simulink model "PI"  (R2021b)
settings: Solver=VariableStepAuto  StartTime=0.0  StopTime=5  RelTol=1e-3
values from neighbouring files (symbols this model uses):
  a = 0.27    [CompareGazeboSimulink.m]    (also in RobotModel.m)
  b = 0.31    [CompareGazeboSimulink.m]    (also in RobotModel.m)
  desired_ang = 1    [RobotModel.m]
  desired_vel = 2    [RobotModel.m]
  Dflag = 1    [RobotModel.m]
  distAng = 0    [RobotModel.m]
  distVel = 0    [RobotModel.m]
  fro = 0.02    [CompareGazeboSimulink.m]    (also in RobotModel.m)
  fsl = 0.8    [CompareGazeboSimulink.m]    (also in RobotModel.m)
  fsly = 0.8    [CompareGazeboSimulink.m]    (also in RobotModel.m)
  I = (1/12)*m*((2*t)^2 + 0.12^2) + 1.5    (= 2.384)    [CompareGazeboSimulink.m]    (also in RobotModel.m = 0.866666666667)
  Iflag = 1    [RobotModel.m]
  K = 22    [RobotModel.m]
  ko = 0    [CompareGazeboSimulink.m]    (also in RobotModel.m = 0.25)
  kt = 0.58    [CompareGazeboSimulink.m]    (also in RobotModel.m)
  m = 51    [CompareGazeboSimulink.m]    (also in RobotModel.m = 50)
  mdy = 10    [CompareGazeboSimulink.m]    (also in RobotModel.m)
  mst = 10    [CompareGazeboSimulink.m]    (also in RobotModel.m)
  N = 0    [RobotModel.m]
  r = 0.19    [CompareGazeboSimulink.m]    (also in RobotModel.m)
  T_vel_variance = 0.0005    [RobotModel.m]
  Td = 0.0125    [RobotModel.m]
  Th0 = 0    [CompareGazeboSimulink.m]    (also in RobotModel.m = 0.9714)
  Th_vel0 = 0    [CompareGazeboSimulink.m]    (also in RobotModel.m)
  Ti = 0.1    [RobotModel.m]
  Ts = 0.01    [CompareGazeboSimulink.m]    (also in RobotModel.m = 0.05)
  X0 = 0    [CompareGazeboSimulink.m]    (also in RobotModel.m)
  x_vel0 = 0    [CompareGazeboSimulink.m]    (also in RobotModel.m)
  x_vel_variance = 0.0005    [RobotModel.m]
  Y0 = 0    [CompareGazeboSimulink.m]    (also in RobotModel.m = 2.5)

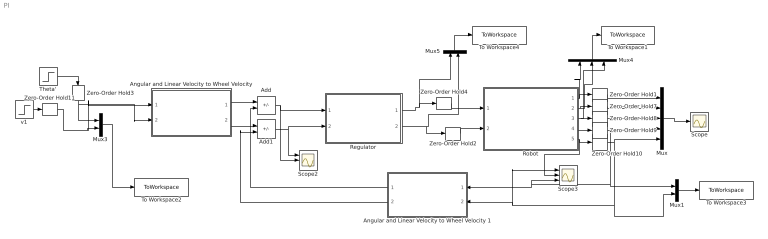
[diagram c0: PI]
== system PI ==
  Add : Sum  Inputs=+-
  Add1 : Sum  Inputs=+-
  Angular and Linear Velocity to Wheel Velocity : Subsystem
  Angular and Linear Velocity to Wheel Velocity 1 : Subsystem
  Mux : Mux  Inputs=5
  Mux1 : Mux  Inputs=2
  Mux3 : Mux  Inputs=2
  Mux4 : Mux  Inputs=3
  Mux5 : Mux  Inputs=2
  Regulator : Subsystem
  Robot : Subsystem
  Scope : Scope
  Scope2 : Scope  NumInputPorts=3
  Scope3 : Scope  NumInputPorts=3
  Theta' : Step  After=desired_ang  SampleTime=0
  To Workspace1 : ToWorkspace  VariableName=ActualPos  SaveFormat=Timeseries  SampleTime=-1
  To Workspace2 : ToWorkspace  VariableName=DesiredVel  SaveFormat=Timeseries  SampleTime=-1
  To Workspace3 : ToWorkspace  VariableName=ActualVel  SaveFormat=Timeseries  SampleTime=-1
  To Workspace4 : ToWorkspace  VariableName=Forces  SaveFormat=Timeseries  SampleTime=-1
  Zero-Order Hold{1..4,7..11} (9 alike) : ZeroOrderHold  SampleTime=Ts
  v1 : Step  After=desired_vel  SampleTime=0
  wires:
  Zero-Order Hold3/1 -> Mux3/1, Angular and Linear Velocity to Wheel Velocity/2(Angular Velocity)
  Zero-Order Hold11/1 -> Angular and Linear Velocity to Wheel Velocity/1(Linear Velocity), Mux3/2
  Zero-Order Hold2/1 -> Robot/2(Right Force)
  Zero-Order Hold4/1 -> Robot/1(Left Force)
  Robot/5(v) -> Scope3/2, Zero-Order Hold10/1
  Robot/3(Theta) -> Mux4/3, Zero-Order Hold8/1
  Robot/2(Y) -> Mux4/2, Zero-Order Hold7/1
  v1/1 -> Zero-Order Hold11/1
  Mux5/1 -> To Workspace4/1
  Mux1/1 -> To Workspace3/1
  Regulator/2(Right force action) -> Mux5/2, Zero-Order Hold2/1
  Add/1 -> Scope2/2, Regulator/1(wl)
  Angular and Linear Velocity to Wheel Velocity/2("wr ") -> Add1/1
  Robot/1(X) -> Mux4/1, Zero-Order Hold1/1
  Angular and Linear Velocity to Wheel Velocity/1(wl) -> Add/1
  Zero-Order Hold8/1 -> Mux/3
  Robot/4(Theta') -> Zero-Order Hold9/1
  Mux3/1 -> To Workspace2/1
  Add1/1 -> Scope2/1, Regulator/2(wr)
  Mux4/1 -> To Workspace1/1
  Angular and Linear Velocity to Wheel Velocity 1/2("wr ") -> Add1/2
  Zero-Order Hold1/1 -> Mux/1
  Zero-Order Hold7/1 -> Mux/2
  Zero-Order Hold10/1 -> Mux1/2, Scope3/1, Angular and Linear Velocity to Wheel Velocity 1/2(Linear Velocity), Mux/5
  Angular and Linear Velocity to Wheel Velocity 1/1(wl) -> Add/2
  Zero-Order Hold9/1 -> Mux1/1, Scope3/3, Angular and Linear Velocity to Wheel Velocity 1/1(Angular Velocity), Mux/4
  Regulator/1(Left Force action) -> Mux5/1, Zero-Order Hold4/1
  Theta'/1 -> Zero-Order Hold3/1
  Mux/1 -> Scope/1

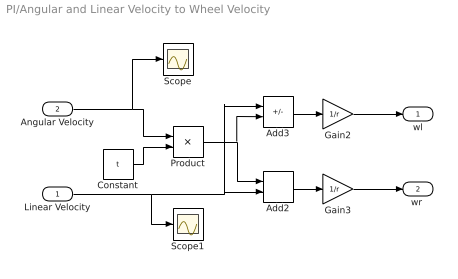
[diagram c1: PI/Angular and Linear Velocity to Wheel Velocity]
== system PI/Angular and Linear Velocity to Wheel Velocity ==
  Linear Velocity : Inport
  Angular Velocity : Inport  Port=2
  Add2 : Sum
  Add3 : Sum  Inputs=+-
  Constant : Constant  Value=t
  Gain2 : Gain  Gain=1/r
  Gain3 : Gain  Gain=1/r
  Product : Product
  Scope : Scope
  Scope1 : Scope
  wl : Outport
  "wr " : Outport  Port=2
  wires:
  Gain2/1 -> wl/1
  Linear Velocity/1 -> Scope1/1, Add2/2, Add3/1
  Gain3/1 -> "wr "/1
  Product/1 -> Add3/2, Add2/1
  Constant/1 -> Product/2
  Add3/1 -> Gain2/1
  Add2/1 -> Gain3/1
  Angular Velocity/1 -> Scope/1, Product/1

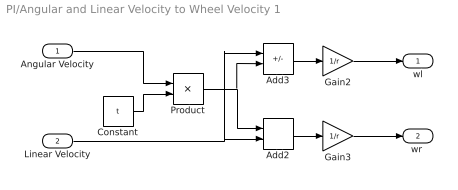
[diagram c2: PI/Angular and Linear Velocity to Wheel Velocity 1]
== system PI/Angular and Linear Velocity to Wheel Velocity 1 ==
  Angular Velocity : Inport
  Linear Velocity : Inport  Port=2
  Add2 : Sum
  Add3 : Sum  Inputs=+-
  Constant : Constant  Value=t
  Gain2 : Gain  Gain=1/r
  Gain3 : Gain  Gain=1/r
  Product : Product
  wl : Outport
  "wr " : Outport  Port=2
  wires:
  Angular Velocity/1 -> Product/1
  Add2/1 -> Gain3/1
  Add3/1 -> Gain2/1
  Constant/1 -> Product/2
  Product/1 -> Add2/1, Add3/2
  Gain3/1 -> "wr "/1
  Linear Velocity/1 -> Add3/1, Add2/2
  Gain2/1 -> wl/1

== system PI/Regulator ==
  wl : Inport
  wr : Inport  Port=2
  PSDN : Subsystem
  PSDN1 : Subsystem
  Left Force action : Outport
  Right force action : Outport  Port=2
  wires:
  wl/1 -> PSDN/1(wl)
  PSDN/1(Left Force action) -> Left Force action/1
  wr/1 -> PSDN1/1(wr)
  PSDN1/1(Right force action) -> Right force action/1

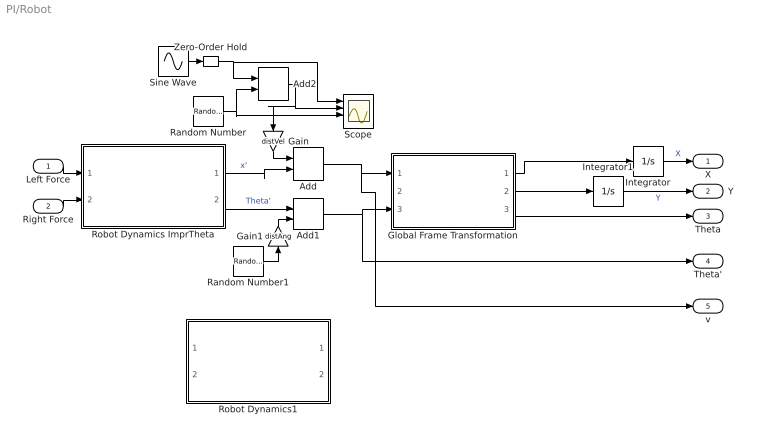
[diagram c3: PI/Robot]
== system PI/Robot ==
  Left Force : Inport
  Right Force : Inport  Port=2
  Add : Sum
  Add1 : Sum
  Add2 : Sum
  Gain : Gain  Gain=distVel
  Gain1 : Gain  Gain=distAng
  Global Frame Transformation : Subsystem
  Integrator : Integrator  InitialCondition=X0
  Integrator1 : Integrator  InitialCondition=Y0
  Random Number : RandomNumber  Variance=x_vel_variance  SampleTime=0.2
  Random Number1 : RandomNumber  Variance=T_vel_variance  SampleTime=0.2
  Robot Dynamics ImprTheta : Subsystem
  Robot Dynamics1 : Subsystem  Commented=on
  Scope : Scope  NumInputPorts=4
  Sine Wave : Sin  Amplitude=0.1*desired_vel  Frequency=0.5  SampleTime=0
  Zero-Order Hold : ZeroOrderHold  SampleTime=0.25
  X : Outport
  Y : Outport  Port=2
  Theta : Outport  Port=3
  Theta' : Outport  Port=4
  v : Outport  Port=5
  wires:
  Random Number/1 -> Add2/2, Scope/3
  Add2/1 -> Gain/1, Scope/2
  Gain/1 -> Add/1
  Sine Wave/1 -> Zero-Order Hold/1
  Add/1 -> v/1, Global Frame Transformation/1(x')
  Add1/1 -> Theta'/1, Global Frame Transformation/3(Theta')
  Random Number1/1 -> Gain1/1
  Left Force/1 -> Robot Dynamics ImprTheta/1(Left Force)
  Gain1/1 -> Add1/2
  Integrator1/1 -> Y/1  "Y"
  Zero-Order Hold/1 -> Scope/1, Add2/1
  Robot Dynamics ImprTheta/1(x') -> Add/2  "x'"
  Global Frame Transformation/2(Y') -> Integrator1/1
  Integrator/1 -> X/1  "X"
  Right Force/1 -> Robot Dynamics ImprTheta/2(Right Force)
  Global Frame Transformation/1(X') -> Integrator/1
  Global Frame Transformation/3(Theta) -> Theta/1
  Robot Dynamics ImprTheta/2(Theta') -> Add1/1  "Theta'"

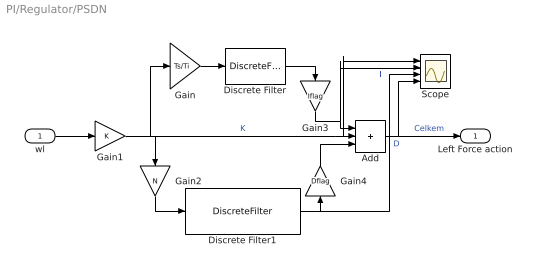
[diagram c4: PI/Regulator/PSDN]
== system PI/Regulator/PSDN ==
  wl : Inport
  Add : Sum  Inputs=3
  Discrete Filter : DiscreteFilter  Numerator=[0 1]  Denominator=[1 -1]
  Discrete Filter1 : DiscreteFilter  Numerator=[1 -1]  Denominator=[1 -exp(-Ts*N/Td)]
  Gain : Gain  Gain=Ts/Ti
  Gain1 : Gain  Gain=K
  Gain2 : Gain  Gain=N
  Gain3 : Gain  Gain=Iflag
  Gain4 : Gain  Gain=Dflag
  Scope : Scope  NumInputPorts=4
  Left Force action : Outport
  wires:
  Discrete Filter/1 -> Gain3/1
  Discrete Filter1/1 -> Scope/3, Gain4/1  "D"
  wl/1 -> Gain1/1
  Add/1 -> Left Force action/1, Scope/4  "Celkem"
  Gain/1 -> Discrete Filter/1
  Gain1/1 -> Gain2/1, Gain/1, Scope/1, Add/2  "K"
  Gain2/1 -> Discrete Filter1/1
  Gain3/1 -> Scope/2, Add/1  "I"
  Gain4/1 -> Add/3

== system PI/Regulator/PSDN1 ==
  wr : Inport
  Add : Sum  Inputs=3
  Discrete Filter : DiscreteFilter  Numerator=[0 1]  Denominator=[1 -1]
  Discrete Filter1 : DiscreteFilter  Numerator=[1 -1]  Denominator=[1 -exp(-Ts*N/Td)]
  Gain : Gain  Gain=Ts/Ti
  Gain1 : Gain  Gain=K
  Gain2 : Gain  Gain=N
  Gain3 : Gain  Gain=Iflag
  Gain4 : Gain  Gain=Dflag
  Right force action : Outport
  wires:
  Gain2/1 -> Discrete Filter1/1
  Gain1/1 -> Add/2, Gain/1, Gain2/1
  Gain/1 -> Discrete Filter/1
  Add/1 -> Right force action/1
  wr/1 -> Gain1/1
  Discrete Filter1/1 -> Gain4/1
  Discrete Filter/1 -> Gain3/1
  Gain3/1 -> Add/1
  Gain4/1 -> Add/3

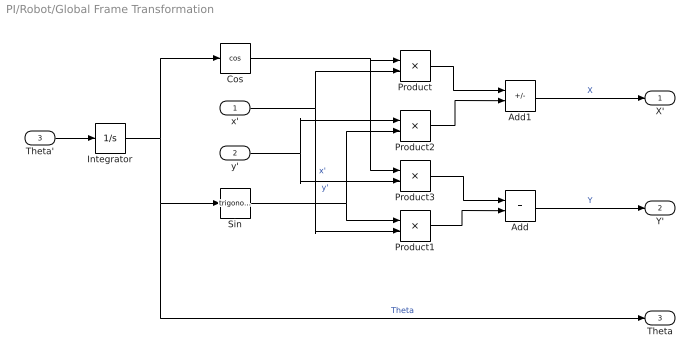
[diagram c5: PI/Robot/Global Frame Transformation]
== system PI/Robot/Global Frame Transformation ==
  x' : Inport
  y' : Inport  Port=2
  Theta' : Inport  Port=3
  Add : Sum
  Add1 : Sum  Inputs=+-
  Cos : Trigonometry  Operator=cos
  Integrator : Integrator  InitialCondition=Th0
  Product{,1..3} (4 alike) : Product
  Sin : Trigonometry
  X' : Outport
  Y' : Outport  Port=2
  Theta : Outport  Port=3
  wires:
  Add/1 -> Y'/1  "Y"
  Integrator/1 -> Theta/1, Sin/1, Cos/1  "Theta"
  Product1/1 -> Add/2
  x'/1 -> Product/2, Product1/2  "x'"
  Sin/1 -> Product1/1, Product2/2
  Product2/1 -> Add1/2
  Product3/1 -> Add/1
  Product/1 -> Add1/1
  Cos/1 -> Product/1, Product3/1
  y'/1 -> Product3/2, Product2/1  "y'"
  Add1/1 -> X'/1  "X"
  Theta'/1 -> Integrator/1

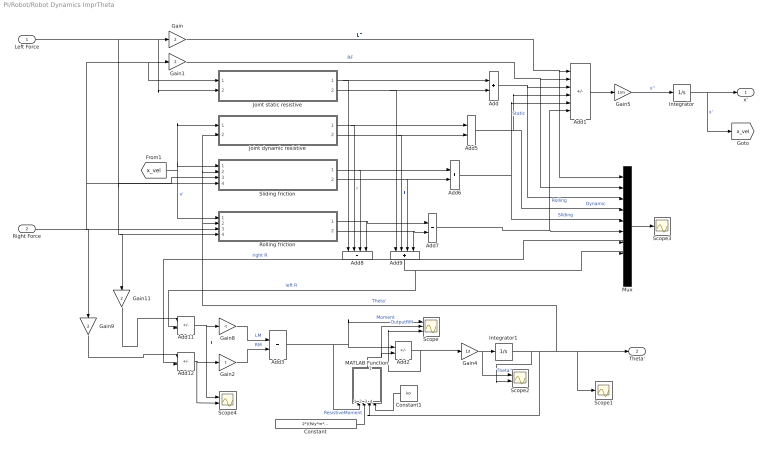
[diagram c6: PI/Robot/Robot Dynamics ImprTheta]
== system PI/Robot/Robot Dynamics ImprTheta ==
  Left Force : Inport
  Right Force : Inport  Port=2
  Add{,3,5..7} (5 alike) : Sum
  Add1 : Sum  Inputs=++----
  Add11 : Sum  Inputs=+-
  Add12 : Sum  Inputs=+-
  Add2 : Sum  Inputs=+-
  Add8 : Sum  Inputs=++++
  Add9 : Sum  Inputs=++++
  Constant : Constant  Value=2*((fsly*m*9.81)/(a+b))*a*b*kt
  Constant1 : Constant  Value=ko
  Gain{,1,9,11} (4 alike) : Gain  Gain=2
  Gain2 : Gain  Gain=t
  Gain4 : Gain  Gain=1/I
  Gain5 : Gain  Gain=1/m
  Gain8 : Gain  Gain=-t
  Integrator : Integrator  InitialCondition=x_vel0
  Integrator1 : Integrator  InitialCondition=Th_vel0
  Joint dynamic resistive : Subsystem
  Joint static resistive : Subsystem
  MATLAB Function : MATLAB Function  TreatAsAtomicUnit=on
  Mux : Mux  Inputs=10
  Rolling friction : Subsystem
  Scope : Scope  NumInputPorts=3
  Scope1 : Scope
  Scope2 : Scope  NumInputPorts=2
  Scope3 : Scope
  Scope4 : Scope  NumInputPorts=2
  Sliding friction : Subsystem
  x' : Outport
  Theta' : Outport  Port=2
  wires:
  Gain4/1 -> Scope2/1, Integrator1/1  "Theta''"
  Integrator1/1 -> Scope2/2, Sliding friction/2(Theta'), Joint dynamic resistive/2(Theta'), Rolling friction/2(Theta'), Scope1/1, Theta'/1, MATLAB Function/3(Omega)  "Theta'"
  Gain1/1 -> Mux/2, Add1/2  "RF"
  Add1/1 -> Gain5/1
  Gain5/1 -> Integrator/1  "x''"
  Integrator/1 -> x'/1, [x_vel]  "x'"
  [x_vel] -> Joint dynamic resistive/1("Local Long Velocity "), Sliding friction/1(Local longitudal velocity), Rolling friction/1(Local longitudal velocity)  "x'"
  Joint static resistive/2(Static Resistive Force Left) -> Add9/1, Add/2
  Joint dynamic resistive/1(Dynamic Resistive Force Right) -> Add8/2, Add5/1  "r"
  Joint dynamic resistive/2(Dynamic Resistive Force Left) -> Add9/2, Add5/2  "l"
  Sliding friction/1(Friction Right Force) -> Add8/3, Add6/1
  Sliding friction/2(Friction Left Force) -> Add9/3, Add6/2
  Rolling friction/1(Friction Right Force) -> Add8/4, Add7/1
  Rolling friction/2(Friction Left Force) -> Add9/4, Add7/2
  Add/1 -> Add1/3, Mux/3  "Static"
  Add6/1 -> Add1/5, Mux/5  "Sliding"
  Add7/1 -> Mux/6, Add1/6  "Rolling"
  Add5/1 -> Mux/4, Add1/4  "Dynamic"
  Add9/1 -> Add11/2, Mux/8  "left R"
  Add8/1 -> Add12/2, Mux/7  "right R"
  Mux/1 -> Scope3/1
  Add11/1 -> Scope4/1, Gain8/1  "LL"
  Add12/1 -> Scope4/2, Gain2/1
  Gain9/1 -> Add12/1
  Gain11/1 -> Add11/1
  Gain8/1 -> Add3/1  "LM"
  Gain2/1 -> Add3/2  "RM"
  Gain/1 -> Mux/1, Add1/1  "LF"
  Joint static resistive/1(Static Resistive Force Right) -> Add8/1, Add/1
  Add2/1 -> Scope/3, Gain4/1
  Add3/1 -> Scope/1, Add2/1, MATLAB Function/1(Moment)  "Moment"
  MATLAB Function/1(y) -> Scope/2, Add2/2  "OutputRM"
  Constant/1 -> MATLAB Function/2(ResistiveMoment)  "ResistiveMoment"
  Left Force/1 -> Gain11/1, Rolling friction/4(Fl), Sliding friction/4(Fl), Joint static resistive/2("Fl "), Gain/1
  Right Force/1 -> Gain9/1, Rolling friction/3(Fr), Sliding friction/3(Fr), Joint static resistive/1(Fr), Gain1/1
  Constant1/1 -> MATLAB Function/4(ko)

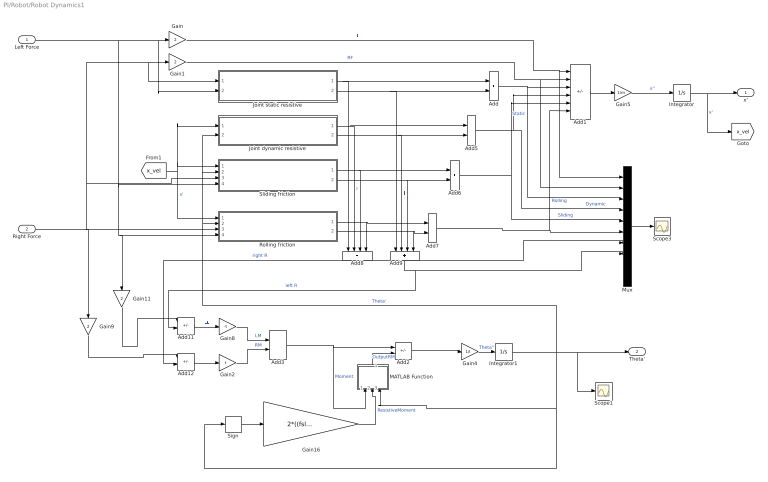
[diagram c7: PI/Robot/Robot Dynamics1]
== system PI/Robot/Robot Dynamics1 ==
  Left Force : Inport
  Right Force : Inport  Port=2
  Add{,3,5..7} (5 alike) : Sum
  Add1 : Sum  Inputs=++----
  Add11 : Sum  Inputs=+-
  Add12 : Sum  Inputs=+-
  Add2 : Sum  Inputs=+-
  Add8 : Sum  Inputs=++++
  Add9 : Sum  Inputs=++++
  Gain{,1,9,11} (4 alike) : Gain  Gain=2
  Gain16 : Gain  Gain=2*((fsly*m*9.81)/(a+b))*a*b
  Gain2 : Gain  Gain=t
  Gain4 : Gain  Gain=1/I
  Gain5 : Gain  Gain=1/m
  Gain8 : Gain  Gain=-t
  Integrator : Integrator  InitialCondition=x_vel0
  Integrator1 : Integrator  InitialCondition=Th_vel0
  Joint dynamic resistive : Subsystem
  Joint static resistive : Subsystem
  MATLAB Function : MATLAB Function  TreatAsAtomicUnit=on
  Mux : Mux  Inputs=10
  Rolling friction : Subsystem
  Scope1 : Scope
  Scope3 : Scope
  Sign : Signum
  Sliding friction : Subsystem
  x' : Outport
  Theta' : Outport  Port=2
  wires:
  Right Force/1 -> Rolling friction/3(Fr), Sliding friction/3(Fr), Joint static resistive/1(Fr), Gain1/1, Gain9/1
  Gain4/1 -> Integrator1/1  "Theta''"
  Integrator1/1 -> Sliding friction/2(Theta'), Joint dynamic resistive/2(Theta'), Rolling friction/2(Theta'), MATLAB Function/3(Omega), Sign/1, Scope1/1, Theta'/1  "Theta'"
  Left Force/1 -> Rolling friction/4(Fl), Gain11/1, Sliding friction/4(Fl), Joint static resistive/2("Fl "), Gain/1
  Gain1/1 -> Mux/2, Add1/2  "RF"
  Add1/1 -> Gain5/1
  Gain5/1 -> Integrator/1  "x''"
  Integrator/1 -> x'/1, [x_vel]  "x'"
  [x_vel] -> Joint dynamic resistive/1("Local Long Velocity "), Sliding friction/1(Local longitudal velocity), Rolling friction/1(Local longitudal velocity)  "x'"
  Joint static resistive/2(Static Resistive Force Left) -> Add9/1, Add/2
  Joint dynamic resistive/1(Dynamic Resistive Force Right) -> Add8/2, Add5/1  "r"
  Joint dynamic resistive/2(Dynamic Resistive Force Left) -> Add9/2, Add5/2  "l"
  Sliding friction/1(Friction Right Force) -> Add8/3, Add6/1
  Sliding friction/2(Friction Left Force) -> Add9/3, Add6/2
  Rolling friction/1(Friction Right Force) -> Add8/4, Add7/1
  Rolling friction/2(Friction Left Force) -> Add9/4, Add7/2
  Add/1 -> Add1/3, Mux/3  "Static"
  Add6/1 -> Add1/5, Mux/5  "Sliding"
  Add7/1 -> Mux/6, Add1/6  "Rolling"
  Add5/1 -> Mux/4, Add1/4  "Dynamic"
  Add9/1 -> Add11/2, Mux/8  "left R"
  Add8/1 -> Add12/2, Mux/7  "right R"
  Mux/1 -> Scope3/1
  Add11/1 -> Gain8/1  "LL"
  Add12/1 -> Gain2/1
  Gain9/1 -> Add12/1
  Gain11/1 -> Add11/1
  Gain8/1 -> Add3/1  "LM"
  Gain2/1 -> Add3/2  "RM"
  Gain/1 -> Mux/1, Add1/1  "LF"
  Joint static resistive/1(Static Resistive Force Right) -> Add8/1, Add/1
  Sign/1 -> Gain16/1
  Add2/1 -> Gain4/1
  Add3/1 -> Add2/1, MATLAB Function/1(Moment)  "Moment"
  MATLAB Function/1(y) -> Add2/2  "OutputRM"
  Gain16/1 -> MATLAB Function/2(ResistiveMoment)  "ResistiveMoment"

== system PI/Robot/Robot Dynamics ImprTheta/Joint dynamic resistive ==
  "Local Long Velocity " : Inport
  Theta' : Inport  Port=2
  Add2 : Sum  Inputs=+-
  Add5 : Sum
  Gain : Gain  Gain=(2*mdy)/(r*r)
  Gain1 : Gain  Gain=(2*mdy)/(r*r)
  Gain4 : Gain  Gain=t
  Scope : Scope  NumInputPorts=3
  Dynamic Resistive Force Right : Outport
  Dynamic Resistive Force Left : Outport  Port=2
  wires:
  Gain/1 -> Dynamic Resistive Force Right/1
  Gain1/1 -> Dynamic Resistive Force Left/1
  Gain4/1 -> Add5/2, Add2/2
  Theta'/1 -> Scope/3, Gain4/1
  Add5/1 -> Scope/2, Gain/1  "vr"
  Add2/1 -> Scope/1, Gain1/1  "vl"
  "Local Long Velocity "/1 -> Add2/1, Add5/1

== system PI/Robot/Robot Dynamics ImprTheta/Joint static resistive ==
  Fr : Inport
  "Fl " : Inport  Port=2
  Fsj : Gain  Gain=2*(mst/r)
  Fsj . : Gain  Gain=2*(mst/r)
  Gain1 : Gain  Gain=1/(mst/r)
  Gain2 : Gain  Gain=1/(mst/r)
  Tanh : Trigonometry  Operator=tanh
  Tanh1 : Trigonometry  Operator=tanh
  Static Resistive Force Right : Outport
  Static Resistive Force Left : Outport  Port=2
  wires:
  Fr/1 -> Gain1/1
  "Fl "/1 -> Gain2/1
  Tanh/1 -> Fsj/1
  Tanh1/1 -> Fsj ./1
  Gain1/1 -> Tanh/1
  Gain2/1 -> Tanh1/1
  Fsj/1 -> Static Resistive Force Right/1
  Fsj ./1 -> Static Resistive Force Left/1

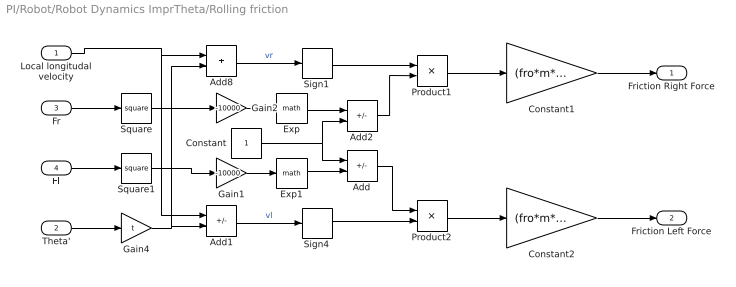
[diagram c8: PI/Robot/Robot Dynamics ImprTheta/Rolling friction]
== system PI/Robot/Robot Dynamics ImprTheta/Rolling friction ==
  Local longitudal velocity : Inport
  Theta' : Inport  Port=2
  Fr : Inport  Port=3
  Fl : Inport  Port=4
  Add : Sum  Inputs=+-
  Add1 : Sum  Inputs=+-
  Add2 : Sum  Inputs=-+
  Add8 : Sum
  Constant : Constant
  Constant1 : Gain  Gain=(fro*m*9.81)/2
  Constant2 : Gain  Gain=(fro*m*9.81)/2
  Exp : Math
  Exp1 : Math
  Gain1 : Gain  Gain=-10000
  Gain2 : Gain  Gain=-10000
  Gain4 : Gain  Gain=t
  Product1 : Product
  Product2 : Product
  Sign1 : Signum
  Sign4 : Signum
  Square : Math  Operator=square
  Square1 : Math  Operator=square
  Friction Right Force : Outport
  Friction Left Force : Outport  Port=2
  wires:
  Sign1/1 -> Product1/1
  Sign4/1 -> Product2/2
  Add8/1 -> Sign1/1  "vr"
  Fl/1 -> Square1/1
  Fr/1 -> Square/1
  Square1/1 -> Gain1/1
  Gain4/1 -> Add1/2, Add8/2
  Theta'/1 -> Gain4/1
  Add1/1 -> Sign4/1  "vl"
  Square/1 -> Gain2/1
  Gain2/1 -> Exp/1
  Gain1/1 -> Exp1/1
  Add2/1 -> Product1/2
  Add/1 -> Product2/1
  Exp1/1 -> Add/2
  Exp/1 -> Add2/1
  Constant/1 -> Add2/2, Add/1
  Local longitudal velocity/1 -> Add1/1, Add8/1
  Product1/1 -> Constant1/1
  Product2/1 -> Constant2/1
  Constant2/1 -> Friction Left Force/1
  Constant1/1 -> Friction Right Force/1

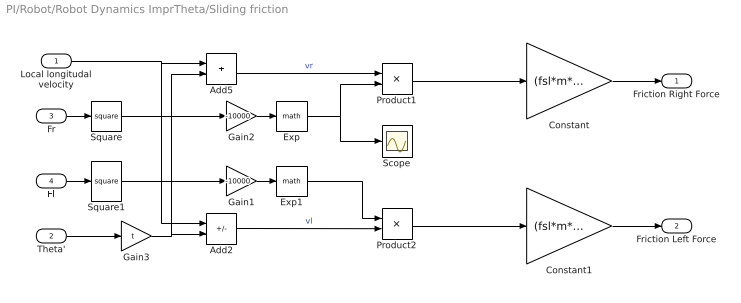
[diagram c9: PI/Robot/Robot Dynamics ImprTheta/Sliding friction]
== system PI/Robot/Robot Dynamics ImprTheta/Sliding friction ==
  Local longitudal velocity : Inport
  Theta' : Inport  Port=2
  Fr : Inport  Port=3
  Fl : Inport  Port=4
  Add2 : Sum  Inputs=+-
  Add5 : Sum
  Constant : Gain  Gain=(fsl*m*9.81)/2
  Constant1 : Gain  Gain=(fsl*m*9.81)/2
  Exp : Math
  Exp1 : Math
  Gain1 : Gain  Gain=-10000
  Gain2 : Gain  Gain=-10000
  Gain3 : Gain  Gain=t
  Product1 : Product
  Product2 : Product
  Scope : Scope
  Square : Math  Operator=square
  Square1 : Math  Operator=square
  Friction Right Force : Outport
  Friction Left Force : Outport  Port=2
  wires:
  Theta'/1 -> Gain3/1
  Gain3/1 -> Add2/2, Add5/2
  Add5/1 -> Product1/1  "vr"
  Add2/1 -> Product2/2  "vl"
  Exp/1 -> Scope/1, Product1/2
  Gain1/1 -> Exp1/1
  Gain2/1 -> Exp/1
  Fr/1 -> Square/1
  Fl/1 -> Square1/1
  Square/1 -> Gain2/1
  Square1/1 -> Gain1/1
  Product1/1 -> Constant/1
  Product2/1 -> Constant1/1
  Exp1/1 -> Product2/1
  Local longitudal velocity/1 -> Add2/1, Add5/1
  Constant/1 -> Friction Right Force/1
  Constant1/1 -> Friction Left Force/1

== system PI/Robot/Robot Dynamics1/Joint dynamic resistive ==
  "Local Long Velocity " : Inport
  Theta' : Inport  Port=2
  Add2 : Sum  Inputs=+-
  Add5 : Sum
  Gain : Gain  Gain=(2*mdy)/(r*r)
  Gain1 : Gain  Gain=(2*mdy)/(r*r)
  Gain4 : Gain  Gain=t
  Scope : Scope  NumInputPorts=3
  Dynamic Resistive Force Right : Outport
  Dynamic Resistive Force Left : Outport  Port=2
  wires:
  Gain/1 -> Dynamic Resistive Force Right/1
  Gain1/1 -> Dynamic Resistive Force Left/1
  Gain4/1 -> Add5/2, Add2/2
  Theta'/1 -> Scope/3, Gain4/1
  Add5/1 -> Scope/2, Gain/1  "vr"
  Add2/1 -> Scope/1, Gain1/1  "vl"
  "Local Long Velocity "/1 -> Add2/1, Add5/1

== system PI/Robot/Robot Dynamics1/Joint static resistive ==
  Fr : Inport
  "Fl " : Inport  Port=2
  Fsj : Gain  Gain=2*(mst/r)
  Fsj . : Gain  Gain=2*(mst/r)
  Gain1 : Gain  Gain=1/(mst/r)
  Gain2 : Gain  Gain=1/(mst/r)
  Tanh : Trigonometry  Operator=tanh
  Tanh1 : Trigonometry  Operator=tanh
  Static Resistive Force Right : Outport
  Static Resistive Force Left : Outport  Port=2
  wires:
  Fr/1 -> Gain1/1
  "Fl "/1 -> Gain2/1
  Tanh/1 -> Fsj/1
  Tanh1/1 -> Fsj ./1
  Gain1/1 -> Tanh/1
  Gain2/1 -> Tanh1/1
  Fsj/1 -> Static Resistive Force Right/1
  Fsj ./1 -> Static Resistive Force Left/1

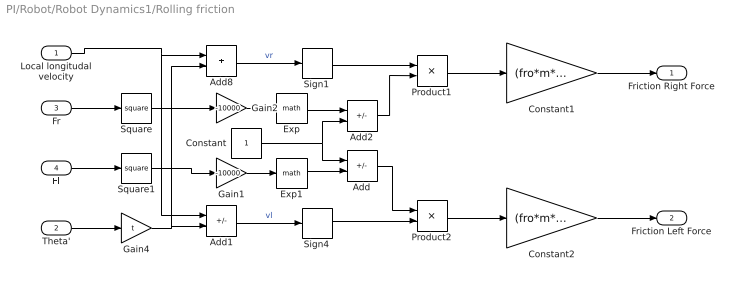
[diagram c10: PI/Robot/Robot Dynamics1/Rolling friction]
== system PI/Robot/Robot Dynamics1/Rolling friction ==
  Local longitudal velocity : Inport
  Theta' : Inport  Port=2
  Fr : Inport  Port=3
  Fl : Inport  Port=4
  Add : Sum  Inputs=+-
  Add1 : Sum  Inputs=+-
  Add2 : Sum  Inputs=-+
  Add8 : Sum
  Constant : Constant
  Constant1 : Gain  Gain=(fro*m*9.81)/2
  Constant2 : Gain  Gain=(fro*m*9.81)/2
  Exp : Math
  Exp1 : Math
  Gain1 : Gain  Gain=-10000
  Gain2 : Gain  Gain=-10000
  Gain4 : Gain  Gain=t
  Product1 : Product
  Product2 : Product
  Sign1 : Signum
  Sign4 : Signum
  Square : Math  Operator=square
  Square1 : Math  Operator=square
  Friction Right Force : Outport
  Friction Left Force : Outport  Port=2
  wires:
  Sign1/1 -> Product1/1
  Sign4/1 -> Product2/2
  Add8/1 -> Sign1/1  "vr"
  Fl/1 -> Square1/1
  Fr/1 -> Square/1
  Square1/1 -> Gain1/1
  Gain4/1 -> Add1/2, Add8/2
  Theta'/1 -> Gain4/1
  Add1/1 -> Sign4/1  "vl"
  Square/1 -> Gain2/1
  Gain2/1 -> Exp/1
  Gain1/1 -> Exp1/1
  Add2/1 -> Product1/2
  Add/1 -> Product2/1
  Exp1/1 -> Add/2
  Exp/1 -> Add2/1
  Constant/1 -> Add2/2, Add/1
  Local longitudal velocity/1 -> Add1/1, Add8/1
  Product1/1 -> Constant1/1
  Product2/1 -> Constant2/1
  Constant2/1 -> Friction Left Force/1
  Constant1/1 -> Friction Right Force/1

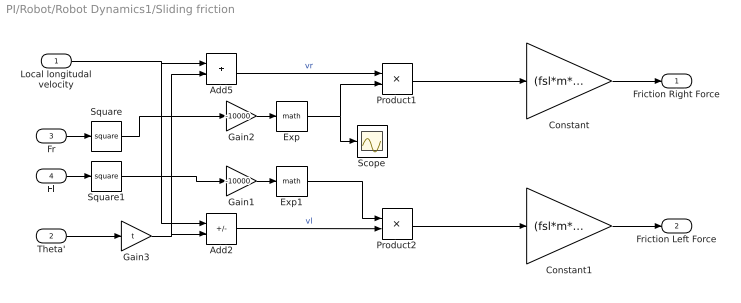
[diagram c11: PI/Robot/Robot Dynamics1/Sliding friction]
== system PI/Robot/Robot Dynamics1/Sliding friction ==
  Local longitudal velocity : Inport
  Theta' : Inport  Port=2
  Fr : Inport  Port=3
  Fl : Inport  Port=4
  Add2 : Sum  Inputs=+-
  Add5 : Sum
  Constant : Gain  Gain=(fsl*m*9.81)/2
  Constant1 : Gain  Gain=(fsl*m*9.81)/2
  Exp : Math
  Exp1 : Math
  Gain1 : Gain  Gain=-10000
  Gain2 : Gain  Gain=-10000
  Gain3 : Gain  Gain=t
  Product1 : Product
  Product2 : Product
  Scope : Scope
  Square : Math  Operator=square
  Square1 : Math  Operator=square
  Friction Right Force : Outport
  Friction Left Force : Outport  Port=2
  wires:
  Theta'/1 -> Gain3/1
  Gain3/1 -> Add2/2, Add5/2
  Add5/1 -> Product1/1  "vr"
  Add2/1 -> Product2/2  "vl"
  Exp/1 -> Scope/1, Product1/2
  Gain1/1 -> Exp1/1
  Gain2/1 -> Exp/1
  Fr/1 -> Square/1
  Fl/1 -> Square1/1
  Square/1 -> Gain2/1
  Square1/1 -> Gain1/1
  Product1/1 -> Constant/1
  Product2/1 -> Constant1/1
  Exp1/1 -> Product2/1
  Local longitudal velocity/1 -> Add2/1, Add5/1
  Constant/1 -> Friction Right Force/1
  Constant1/1 -> Friction Left Force/1

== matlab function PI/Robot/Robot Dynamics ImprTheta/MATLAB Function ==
function y = fcn(Moment, ResistiveMoment, Omega, ko)
    y = Omega*ResistiveMoment;

%     if(abs(Moment) < abs(ResistiveMoment))
%         y = Moment;
%     else
%         y = (ko*Omega + sign(Omega))*ResistiveMoment;
%     end



end

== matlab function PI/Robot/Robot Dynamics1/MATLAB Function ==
function y = fcn(Moment, ResistiveMoment, Omega)
    y = ResistiveMoment;
    
    if(Omega ~= 0)
        if(abs(Moment) < abs(ResistiveMoment))
            y = sign(Omega)*abs(Moment);
        else
            y = ResistiveMoment;
        end
    else
        y = 0;


end
